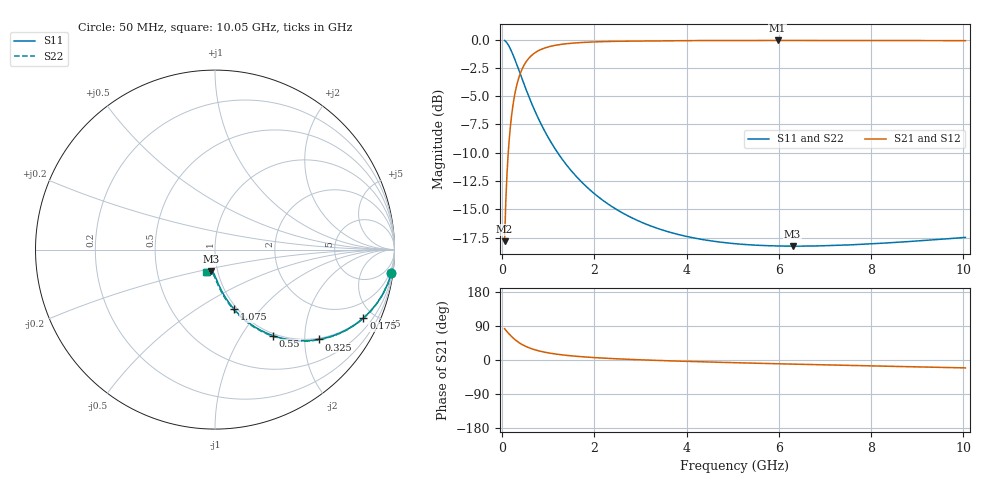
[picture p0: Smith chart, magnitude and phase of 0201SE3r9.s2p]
! AVX Thin Film Operation		Date: August 2001
! Description: Accu-P® Series, Thin Film, SMD, RF Capacitor
! Part Number: 0201YJ3R9ABW
! 50 MHz  -  10.05 GHz
! Serial Measurements
# mhz S db R 50
!	S11		S21		S12		S22
!	dB	Phase	dB	Phase	dB	Phase	dB	Phase
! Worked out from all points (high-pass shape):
!   401 points, 50 MHz to 10.05 GHz, reference 50 ohm
!   highest |S21| = -0.07 dB at 5.975 GHz (marker M1); lowest = -17.8 dB at 50 MHz (marker M2)
!   |S21| within 3 dB of the highest: 383.2 MHz to end of sweep
!   lowest |S11| = -18.3 dB at 6.3 GHz (marker M3), VSWR 1.28, Z = 46.7 - j11.4 ohm
!   |S11| at or under -10 dB: 1.202 GHz to end of sweep
!   |S22| runs from -18.3 to -0.1 dB; largest |S21 - S12| = 0
!   S11 on the Smith chart (normalised r, x): 50 MHz: 1, -15; 175 MHz: 0.97, -4.35; 325 MHz: 0.97, -2.34; 550 MHz: 0.97, -1.39; 1.075 GHz: 0.97, -0.73; 10.05 GHz: 0.89, -0.23
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50  -0.07 -7.5  -17.83 82.5  -17.83 82.5  -0.07 -7.5
75  -0.16 -11.2  -14.40 78.8  -14.40 78.8  -0.16 -11.2
125  -0.43 -18.2  -10.24 71.7  -10.24 71.7  -0.43 -18.3
175  -0.81 -24.8  -7.70 65.1  -7.70 65.1  -0.81 -24.9
250  -1.52 -33.5  -5.32 56.4  -5.32 56.4  -1.52 -33.6
325  -2.32 -40.8  -3.85 49.1  -3.85 49.1  -2.31 -41.0
425  -3.42 -48.6  -2.64 41.2  -2.64 41.2  -3.42 -48.9
550  -4.77 -56.1  -1.77 33.7  -1.77 33.7  -4.77 -56.4
650  -5.77 -60.6  -1.34 29.1  -1.34 29.1  -5.77 -61.0
775  -6.91 -65.1  -1.00 24.6  -1.00 24.6  -6.91 -65.5
1075  -9.20 -72.3  -0.56 17.2  -0.56 17.2  -9.19 -73.0
1350  -10.85 -76.7  -0.38 12.8  -0.38 12.8  -10.85 -77.5
1725  -12.61 -80.7  -0.25 8.6  -0.25 8.6  -12.60 -81.7
2475  -15.01 -85.9  -0.15 3.2  -0.15 3.2  -15.01 -87.3
3400  -16.73 -90.2  -0.10 -1.3  -0.10 -1.3  -16.73 -91.8
4175  -17.55 -93.0  -0.09 -4.2  -0.09 -4.2  -17.55 -94.8
5050  -18.04 -95.8  -0.08 -7.2  -0.08 -7.2  -18.05 -97.7
5975  -18.24 -98.6  -0.07 -9.9  -0.07 -9.9  -18.25 -100.4
6300  -18.26 -99.5  -0.07 -10.9  -0.07 -10.9  -18.26 -101.3
6725  -18.25 -100.7  -0.07 -12.1  -0.07 -12.1  -18.25 -102.5
8400  -17.96 -105.2  -0.08 -16.6  -0.08 -16.6  -17.96 -106.9
10050  -17.49 -109.4  -0.09 -20.8  -0.09 -20.8  -17.49 -111.0
